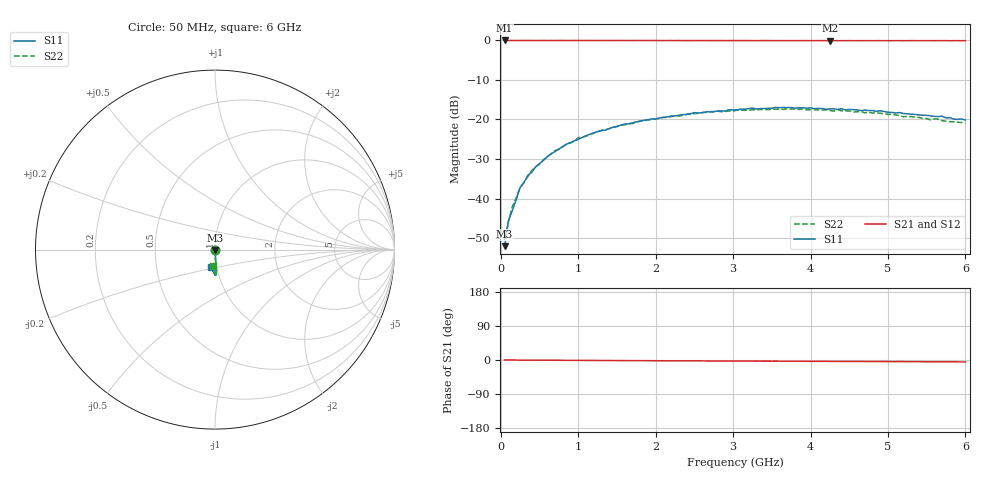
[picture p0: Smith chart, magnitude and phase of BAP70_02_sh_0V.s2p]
!	Created	by	janssen	on	Thu	Dec	12	13:21:33	MET	2002
#	HZ	S	MA	R	50
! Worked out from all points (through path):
!   120 points, 50 MHz to 6 GHz, reference 50 ohm
!   highest |S21| = 0.01 dB at 50 MHz (marker M1); lowest = -0.1 dB at 4.25 GHz (marker M2)
!   lowest |S11| = -52.1 dB at 50 MHz (marker M3), VSWR 1.00, Z = 50 - j0.245 ohm
!   |S11| at or under -10 dB: start of sweep to end of sweep
!   |S22| runs from -50.5 to -17.2 dB; largest |S21 - S12| = 0.0052
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5e7  0.002494 -100.2  1.001 -0.1  0.9997 -0.3  0.00298 -105.1
1e8  0.005203 -99.6  0.9999 -0.1  0.9993 -0.2  0.005132 -90.5
1.5e8  0.007086 -87.2  1 -0.2  0.9991 -0.2  0.007921 -91.7
2.5e8  0.01376 -88.7  0.9999 -0.3  1 -0.3  0.01386 -85.6
3.5e8  0.01969 -86.6  1 -0.3  0.9991 -0.4  0.01889 -82.8
4e8  0.0214 -86.3  1 -0.4  1 -0.4  0.02262 -87.4
4.5e8  0.02511 -84.7  1 -0.5  1 -0.5  0.0252 -85.4
7e8  0.0393 -86.3  0.9998 -0.7  0.9996 -0.7  0.04028 -85.6
8.5e8  0.04879 -85.0  0.9999 -0.8  1 -0.9  0.0487 -86.6
1.05e9  0.05899 -87.2  1 -1.0  1 -1.1  0.05983 -86.8
1.55e9  0.08505 -87.4  0.9995 -1.5  0.9989 -1.5  0.08394 -86.9
2.05e9  0.1044 -86.8  0.9983 -2.0  0.9983 -2.0  0.105 -87.5
2.5e9  0.1222 -86.3  0.9979 -2.3  0.9975 -2.3  0.1187 -87.3
3.05e9  0.1323 -87.0  0.9973 -2.8  0.9961 -2.9  0.1314 -87.0
3.55e9  0.1423 -88.2  0.9948 -3.1  0.9955 -3.3  0.1349 -87.8
4.05e9  0.1371 -89.8  0.9946 -3.5  0.9944 -3.6  0.1332 -88.5
4.25e9  0.1361 -90.6  0.9931 -3.6  0.9932 -3.8  0.13 -89.7
5.05e9  0.1232 -94.9  0.9936 -4.3  0.9921 -4.3  0.1171 -90.7
5.2e9  0.1192 -94.9  0.9935 -4.2  0.9928 -4.4  0.1084 -91.8
5.65e9  0.1091 -97.0  0.9954 -4.8  0.9918 -4.9  0.1011 -94.1
5.7e9  0.1101 -100.5  0.9948 -4.8  0.9926 -4.9  0.09654 -94.4
6e9  0.09846 -102.7  0.9948 -5.0  0.9915 -5.2  0.09001 -98.3
